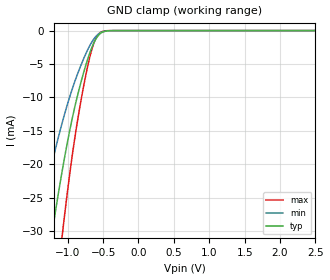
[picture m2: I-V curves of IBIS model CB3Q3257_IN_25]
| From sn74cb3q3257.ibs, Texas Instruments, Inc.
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[Model]   CB3Q3257_IN_25
Model_type  Input
Vinl=0.7
Vinh=1.7
| variable   typ   min   max
C_comp   2.39pF   1.89pF   2.61pF
[Temperature Range]   40   100   -40
| Ambient temperature   25   85   -40
[Voltage range]   2.5   2.3   2.7
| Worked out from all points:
|   GND clamp passes 1 mA (typ) near -0.59 V on its own axis
[GND Clamp]
| CB3Q3257_IN_25
|   Voltage   I(typ)   I(min)   I(max)
-5.5V     -472.4mA   -358mA     -596.1mA
-1.43V    -45.98mA   -30.17mA   -67.32mA
-1.21V    -29.57mA   -19.34mA   -43.56mA
-1.075V   -20.82mA   -13.68mA   -30.43mA
-1.06V    -19.92mA   -13.1mA    -29.06mA
-975mV    -15.15mA   -10.04mA   -21.76mA
-905mV    -11.67mA   -7.786mA   -16.46mA
-780mV    -6.479mA   -4.348mA   -8.607mA
-650mV    -2.304mA   -1.56mA    -2.508mA
-550mV    -541.9uA   -406uA     -369.7uA
-350mV    -3.742uA   -5.538uA   -427.8nA
2.5V      96.07pA    415.1pA    20.34pA
